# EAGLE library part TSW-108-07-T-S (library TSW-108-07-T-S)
8 Position, Single Row, Classic PCB Header Strips, 0.100" pitch Source: Datasheet
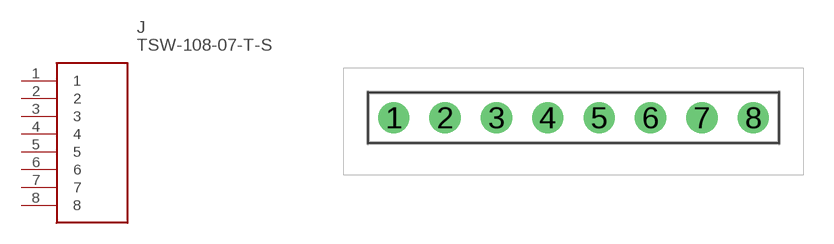
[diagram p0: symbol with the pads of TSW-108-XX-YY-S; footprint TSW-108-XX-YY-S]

Designator prefix J

## TSW-108-07-T-S (Description: 8 Position, Single Row, Classic PCB Header Strips, 0.100&quot; pitch; Height: mm; Manufacturer_Name: SAMTEC; Manufacturer_Part_Number: TSW-108-07-T-S; Mouser_Part_Number: 200-TSW10807TS; Mouser_Price-Stock: https://www.mouser.co.uk/ProductDetail/Samtec/TSW-108-07-T-S?qs=hzq9O0YpnZvsSJKdpkY6dA%3D%3D)  [TSW-108-XX-YY-S]
1  1
2  2
3  3
4  4
5  5
6  6
7  7
8  8

## Footprint TSW-108-XX-YY-S (pad centres in mm)
TSW-108-XX-YY-S
drill 1.02 pad 1.55: 1 0,0; 2 2.54,0; 3 5.08,0; 4 7.62,0; 5 10.16,0; 6 12.7,0; 7 15.24,0; 8 17.78,0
